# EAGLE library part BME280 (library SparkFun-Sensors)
Bosch BME280 &ndash; Combined Humidity and Pressure Sensor The BME280 is as combined digital humidity, pressure and temperature sensor based on proven sensing principles. The sensor module is housed in an extremely compact metal-lid LGA package with a footprint of only 2.5×2.5mm² with a height of 0.93mm. Its small dimensions and its low power consumption allow the implementation in battery driven devices such as handsets, GPS modules or watches. Datasheet SparkFun Products SparkFun Atmospheric Sensor Breakout - BME280 (SEN-13676)
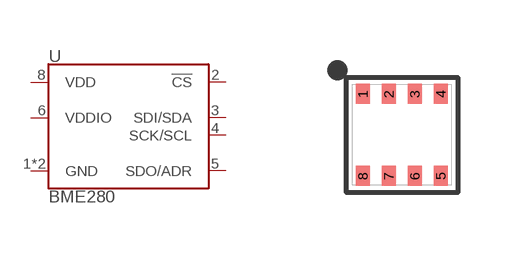
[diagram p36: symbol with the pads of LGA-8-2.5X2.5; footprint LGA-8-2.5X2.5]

Designator prefix U

## BME280 (PROD_ID: IC-13090; VALUE: BME280)  [LGA-8-2.5X2.5]
1  GND
2  !CS
3  SDI/SDA
4  SCK/SCL
5  SDO/ADR
6  VDDIO
7  GND
8  VDD

## Footprint LGA-8-2.5X2.5 (pad centres in mm)
LGA 8-Pin &ndash; 2.5mm x 2.5mm, 0.65mm Pitch Example Datasheet Specifications: Pin Count: 8 Dimensions: 2.5 x 2.5 mm Pitch: 0.65 mm Used by: BME280
smd 0.35 x 0.5: 1 -0.975,1.025; 2 -0.325,1.025; 3 0.325,1.025; 4 0.975,1.025; 5 0.975,-1.025; 6 0.325,-1.025; 7 -0.325,-1.025; 8 -0.975,-1.025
